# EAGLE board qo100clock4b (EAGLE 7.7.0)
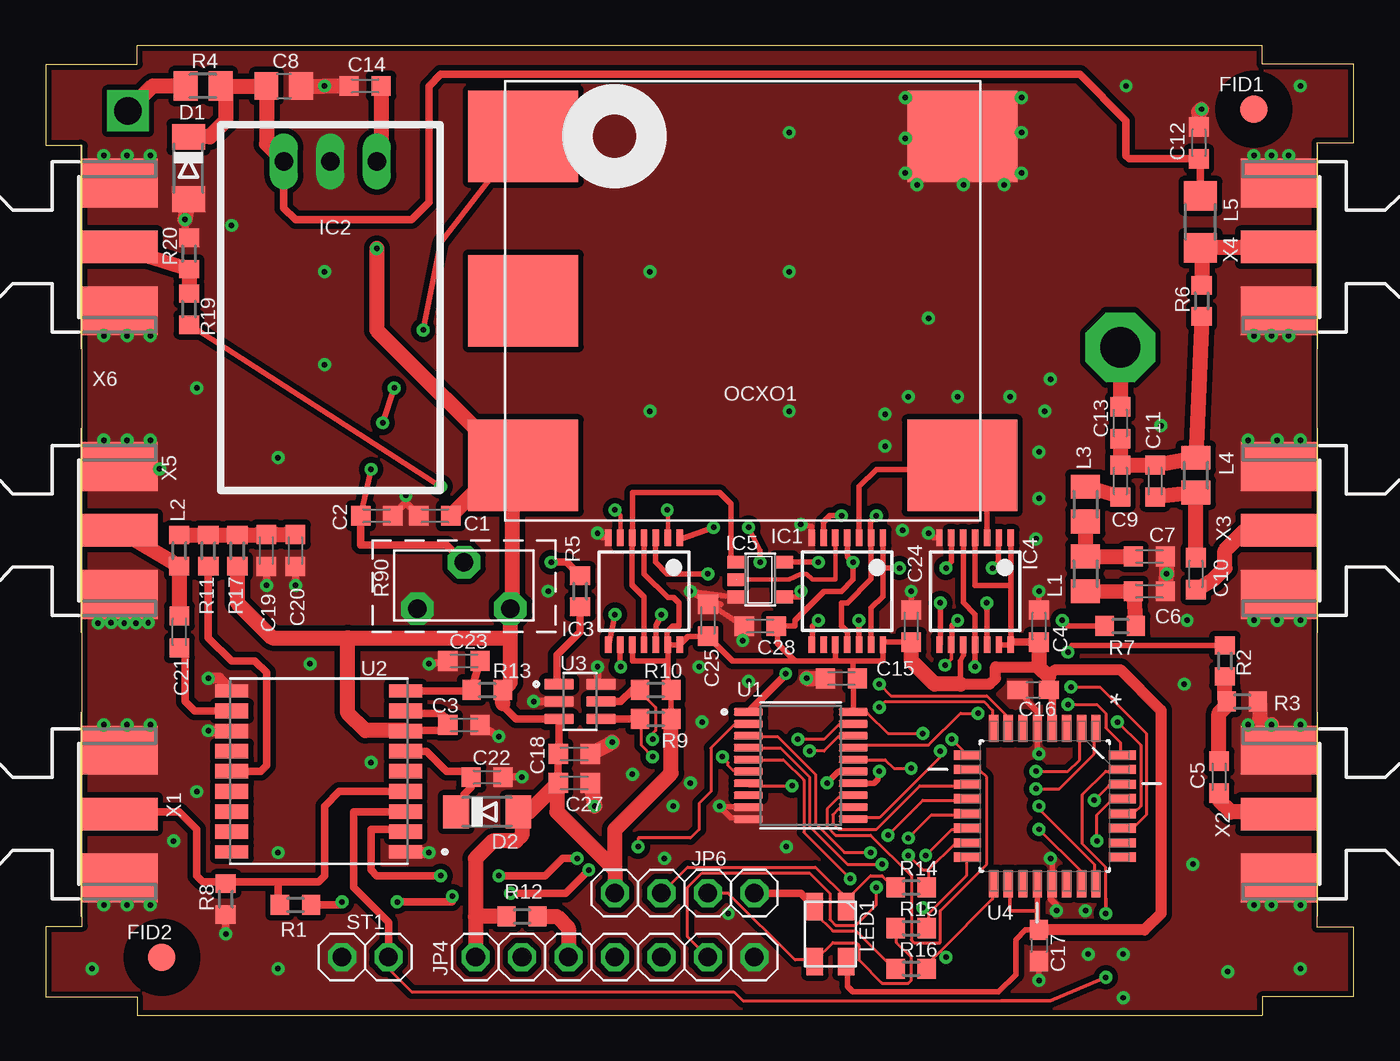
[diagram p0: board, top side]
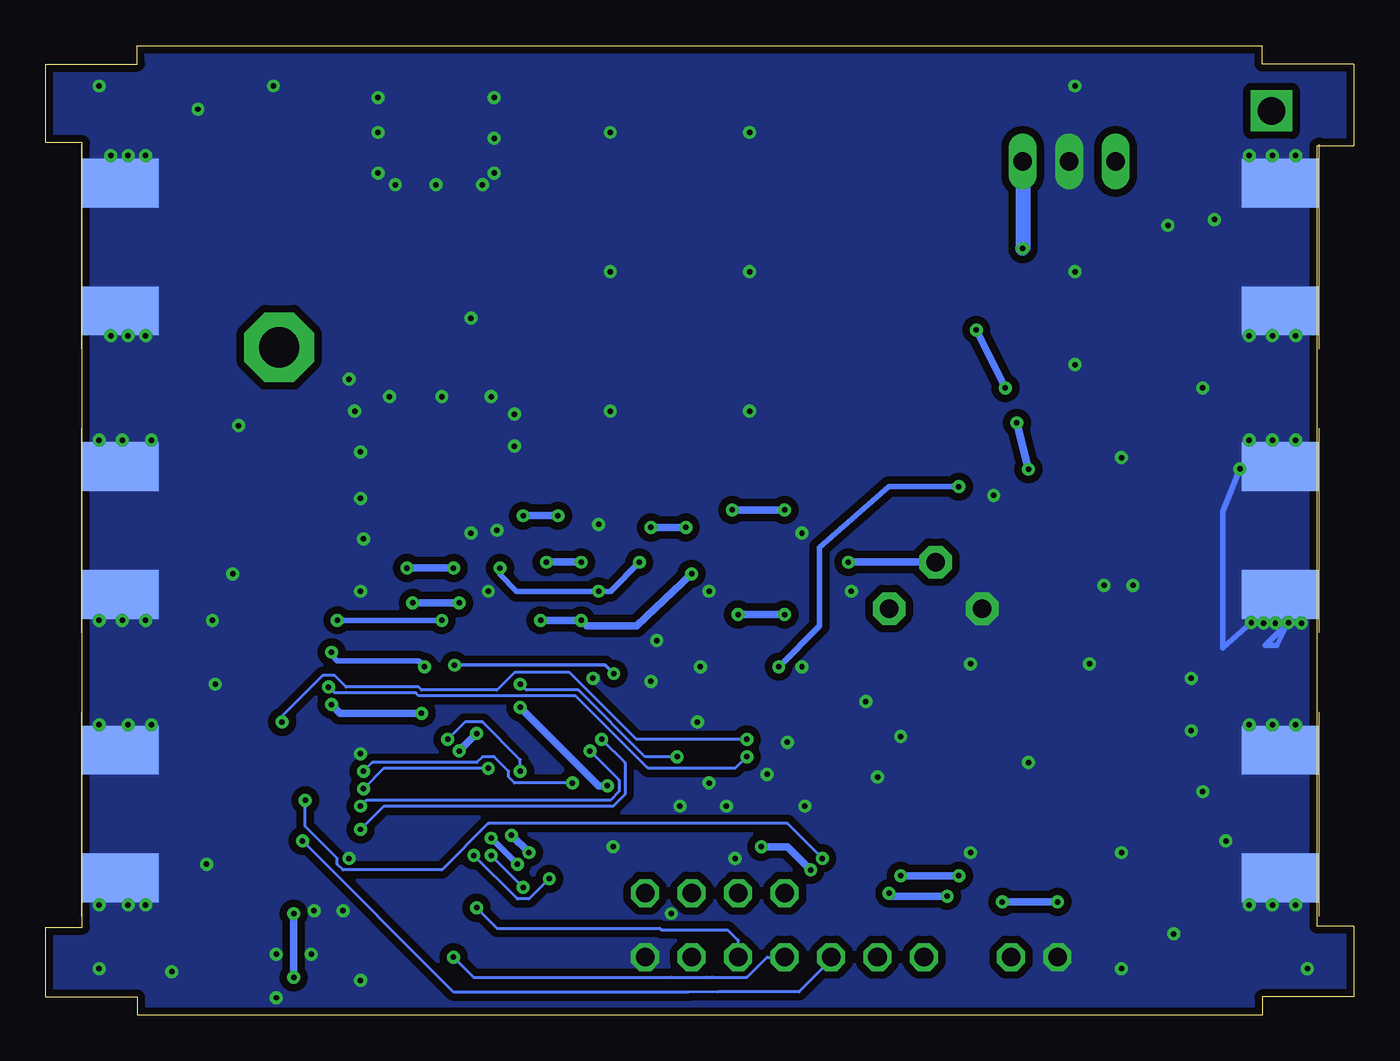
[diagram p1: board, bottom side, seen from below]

Size 71.5 x 53 mm. Coordinates in mm from the lower left corner, seen from the top.
Outline: 5,0 66.5,0 66.5,1 71.5,1 71.5,4.82 69.5,4.82 69.5,47.69 71.5,47.69 71.5,52 66.5,52 66.5,53 5,53 5,52 0,52 0,47.53 2,47.53 2,4.87 0,4.87 0,1 5,1 5,0
Copper layers (1*16): Top 0.035mm / dielectric 1.5mm / Bottom 0.035mm
Design rules "default *": minimum track width 6mil, minimum drill 0.3mm, track to track 6mil, track to pad 6mil, pad to pad 6mil, via to via 6mil, smd to smd 0mil, copper to edge 1mil, drill to drill 8mil, minimum pad ring 10mil, minimum via ring 8mil, stop-mask expansion 4mil, vias tented up to drill 0.51mm, thermal gap 10mil

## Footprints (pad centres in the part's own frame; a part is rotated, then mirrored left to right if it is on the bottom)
C0603K = smd 1.05 x 1.08: 1 -0.875,0; 2 0.875,0
C0805 = smd 1.3 x 1.5: 1 -0.95,0; 2 0.95,0
C0603 = smd 1.1 x 1: 1 -0.85,0; 2 0.85,0
MINIMELF = smd 1.4 x 1.8: A 1.7,0; C -1.7,0
FIDUCIAL = smd 1.5 x 1.5: P$1 0,0
TSSOP14 = smd 0.35 x 0.9: 1 -1.95,-2.925; 2 -1.3,-2.925; 3 -0.65,-2.925; 4 0,-2.925; 5 0.65,-2.925; 6 1.3,-2.925; 7 1.95,-2.925; 8 1.95,2.925; 9 1.3,2.925; 10 0.65,2.925; 11 0,2.925; 12 -0.65,2.925; 13 -1.3,2.925; 14 -1.95,2.925
78SR_SWITCHREG = drill 1.016 long: 1 2.54,0; 2 0,0; 3 -2.54,0
SOT23-5 = smd 0.69 x 0.99: 1 -0.95,-1.29; 2 0,-1.29; 3 0.95,-1.29; 4 0.95,1.3; 5 -0.95,1.3
THICKPIN1,5SQU = drill 1.5 square: P$1 0,0
THICKPIN_OCT = drill 2.2 pad 3.81 octagon: 1 0,0
PINHEAD7X1 = drill 1.016 octagon: 1 -7.62,0; 2 -5.08,0; 3 -2.54,0; 4 0,0; 5 2.54,0; 6 5.08,0; 7 7.62,0
PINHEAD4X1 = drill 1.016 octagon: 1 -5.08,0; 2 -2.54,0; 3 0,0; 4 2.54,0
M0805 = smd 1.3 x 1.6: 1 -0.95,0; 2 0.95,0
R0603 = smd 1 x 1.1: 1 -0.85,0; 2 0.85,0
R1206 = smd 1.6 x 1.803: 1 -1.422,0; 2 1.422,0
PLCC4_WE_LED = smd 1.5 x 0.9: 1 1.51,0.88; 2 1.51,-0.82; 3 -1.49,0.88; 4 -1.49,-0.82
OCXO_2522 = smd 5 x 6: P1 -9,-12; P2 0,-12; P3 9,-12; P4 9,12; P5 -9,12
M2012 = smd 1.3 x 1.6: 1 -0.95,0; 2 0.95,0
MINIPOTI = drill 1.016 pad 1.778 octagon: 1 -2.54,-2.54; 2 2.54,-2.54; 3 0,0
PINHEAD1X2 = drill 1.016 octagon: 1 -1.27,0; 2 1.27,0
SOP65P640X120-20N = smd 1.57 x 0.41: 1 -2.87,2.925; 2 -2.87,2.275; 3 -2.87,1.625; 4 -2.87,0.975; 5 -2.87,0.325; 6 -2.87,-0.325; 7 -2.87,-0.975; 8 -2.87,-1.625; 9 -2.87,-2.275; 10 -2.87,-2.925; 11 2.87,-2.925; 12 2.87,-2.275; 13 2.87,-1.625; 14 2.87,-0.975; 15 2.87,-0.325; 16 2.87,0.325; 17 2.87,0.975; 18 2.87,1.625; 19 2.87,2.275; 20 2.87,2.925
XCVR_MAX-M8C-0 = smd 1.8 x 0.7: 1 -4.75,4.4; 9 -4.75,-4.4; 10 4.75,-4.4; 18 4.75,4.4 | smd 1.8 x 0.8: 2 -4.75,3.3; 3 -4.75,2.2; 4 -4.75,1.1; 5 -4.75,0; 6 -4.75,-1.1; 7 -4.75,-2.2; 8 -4.75,-3.3; 11 4.75,-3.3; 12 4.75,-2.2; 13 4.75,-1.1; 14 4.75,0; 15 4.75,1.1; 16 4.75,2.2; 17 4.75,3.3
SOT95P270X145-6N = smd 1.61 x 0.59: 1 -1.145,0.95; 2 -1.145,0; 3 -1.145,-0.95; 4 1.145,-0.95; 5 1.145,0; 6 1.145,0.95
QFP80P900X900X120-32N = smd 1.473 x 0.508: 1 -4.242,2.794; 2 -4.242,2.007; 3 -4.242,1.194; 4 -4.242,0.406; 5 -4.242,-0.406; 6 -4.242,-1.194; 7 -4.242,-2.007; 8 -4.242,-2.794; 17 4.242,-2.794; 18 4.242,-2.007; 19 4.242,-1.194; 20 4.242,-0.406; 21 4.242,0.406; 22 4.242,1.194; 23 4.242,2.007; 24 4.242,2.794 | smd 0.508 x 1.473: 9 -2.794,-4.242; 10 -2.007,-4.242; 11 -1.194,-4.242; 12 -0.406,-4.242; 13 0.406,-4.242; 14 1.194,-4.242; 15 2.007,-4.242; 16 2.794,-4.242; 25 2.794,4.242; 26 2.007,4.242; 27 1.194,4.242; 28 0.406,4.242; 29 -0.406,4.242; 30 -1.194,4.242; 31 -2.007,4.242; 32 -2.794,4.242
J502-ND-142-0711-821/826 = smd 4.191 x 1.778: 1 2.115,0 | smd 4.191 x 2.667: G@1 2.115,3.495; G@2 2.115,-3.495 | smd 4.191 x 2.667 bottom: G@3 2.115,3.495; G@4 2.115,-3.495

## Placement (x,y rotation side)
C1  100n  [C0603K]  21.27,27.3 180 top
C2  10u  [C0603K]  18.1,27.3 0 top
C3  100n  [C0603K]  22.86,15.88 0 top
C4  100n  [C0603K]  54.29,21.27 90 top
C5  100p  [C0603K]  64.14,13.02 270 top
C6  100p  [C0603K]  60.33,23.18 180 top
C7  100p  [C0603K]  60.33,25.08 180 top
C8  10u  [C0805]  13.02,50.8 0 top
C9  100p  [C0603K]  58.74,29.21 270 top
C10  100n  [C0603K]  62.87,24.13 270 top
C11  100p  [C0603K]  60.64,29.21 90 top
C12  100n  [C0603K]  63.03,47.69 270 top
C13  100p  [C0603K]  58.74,32.38 90 top
C14  10u  [C0603K]  17.46,50.8 180 top
C15  100n  [C0603K]  43.5,18.41 180 top
C16  1u/10  [C0603]  53.98,17.78 180 top
C17  1u/10  [C0603]  54.29,3.81 270 top
C18  100n  [C0603K]  28.89,14.29 0 top
C19  100p  [C0603K]  12.06,25.4 270 top
C20  10u  [C0603K]  13.65,25.4 270 top
C21  100p  [C0603K]  7.3,20.95 270 top
C22  10u  [C0603K]  24.13,13.02 0 top
C23  100n  [C0603K]  22.86,19.37 0 top
C24  100n  [C0603K]  47.31,21.27 90 top
C25  100n  [C0603K]  36.2,21.59 90 top
C27  10u  [C0603K]  28.89,12.7 0 top
C28  100n  [C0603K]  39.05,21.27 0 top
D1  Schottky  [MINIMELF]  7.8,46.31 270 top
D2  Schottky  [MINIMELF]  24.13,11.11 0 top
FID1  FIDUCIAL  [FIDUCIAL]  66.04,49.53 0 top
FID2  FIDUCIAL  [FIDUCIAL]  6.35,3.17 0 top
IC1  74LVC74APW-Q100J  [TSSOP14]  43.81,23.18 180 top
IC2  OKI-78SR-3.3/1.5-W36H-C  [78SR_SWITCHREG]  15.56,46.67 180 top
IC3  74LVC74APW-Q100J  [TSSOP14]  32.7,23.18 180 top
IC4  74LVC74APW-Q100J  [TSSOP14]  50.8,23.18 180 top
IC5  74AHC1G00DBV  [SOT23-5]  39.05,23.81 270 top
JP2  [THICKPIN1,5SQU]  4.49,49.44 90 top
JP3  [THICKPIN_OCT]  58.74,36.51 90 top
JP4  Program  [PINHEAD7X1]  31.11,3.17 0 top
JP6  [PINHEAD4X1]  33.66,6.67 180 top
L1  390nH  [M0805]  56.83,24.13 90 top
L2  47nH  [R0603]  7.3,25.4 90 top
L3  390nH  [M0805]  56.83,27.94 90 top
L4  390nH  [M0805]  62.87,29.53 270 top
L5  4.7uH/1A  [R1206]  63.11,43.37 270 top
LED1  WE:150141M173100  [PLCC4_WE_LED]  42.86,4.45 270 top
OCXO1  ECOC-2522-100.000-3-F-C  [OCXO_2522]  38.1,39.05 270 top
R1  1k  [R0603]  13.65,6.03 180 top
R2  100  [R0603]  64.45,19.37 270 top
R3  100  [R0603]  65.41,17.14 180 top
R4  PTC-fuse 2A  [M2012]  8.61,50.8 0 top
R5  10k  [R0603]  29.21,23.18 90 top
R6  0 Ohms  [R0603]  63.18,39.05 90 top
R7  47  [R0603]  58.74,21.27 0 top
R8  1k  [R0603]  9.84,6.35 90 top
R9  2k2  [R0603]  33.34,16.19 0 top
R10  2k2  [R0603]  33.34,17.78 0 top
R11  10  [R0603]  8.89,25.4 90 top
R12  100k  [R0603]  26.04,5.4 0 top
R13  10k  [R0603]  24.13,17.78 0 top
R14  1k  [R0603]  47.31,6.99 0 top
R15  2k2  [R0603]  47.31,4.76 0 top
R16  2k2  [R0603]  47.31,2.54 0 top
R17  NC  [R0603]  10.48,25.4 90 top
R19  100  [R0603]  7.83,38.6 270 top
R20  100  [R0603]  7.83,41.64 90 top
R90  5k  [MINIPOTI]  22.86,24.77 0 top
ST1  [PINHEAD1X2]  17.46,3.17 0 top
U1  SN74LV8154pwr  [SOP65P640X120-20N]  41.27,13.65 0 top
U2  MAX-8Q  [XCVR_MAX-M8C-0]  14.92,13.34 180 top
U3  MCP4725A0T-E/CH  [SOT95P270X145-6N]  29.21,17.14 0 top
U4  ATMEGA88PB-AU  [QFP80P900X900X120-32N]  54.61,11.43 270 top
X1  SMA  [J502-ND-142-0711-821/826]  1.91,11 0 top
X2  SMA  [J502-ND-142-0711-821/826]  69.53,11 180 top
X3  SMA  [J502-ND-142-0711-821/826]  69.53,26.5 180 top
X4  SMA  [J502-ND-142-0711-821/826]  69.53,42 180 top
X5  GPS-ANT  [J502-ND-142-0711-821/826]  1.91,26.5 0 top
X6  SMA  [J502-ND-142-0711-821/826]  1.91,42 0 top

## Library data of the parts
C1-C25 C27 C28 L1-L5 R1-R17 R19 R20 = rcl
D1 D2 = diode
FID1 FID2 IC2 JP2-JP4 JP6 LED1 R90 ST1 = km
IC1 IC3 IC4 = 74xx-eu
IC5 = 74xx-little-de
OCXO1 = km_HF
U1 = SN74LV8154PWR; AVAILABILITY: In Stock; DESCRIPTION: Dual 16-Bit Binary Counters with 3-State Output Registers 20-TSSOP -40 to 85; MF: Texas Instruments; MP: SN74LV8154PWR; PACKAGE: TSSOP-20 Texas Instruments; PRICE: None; PURCHASE-URL: https://pricing.snapeda.com/search/part/SN74LV8154PWR/?ref=eda
U2 = MAX-M8C-0; AVAILABILITY: In Stock; DESCRIPTION: MAX-M8 RF Receiver BeiDou, Galileo, GLONASS, GNSS, GPS 1.575GHz -167dBm; MF: u-blox; MP: MAX-M8C-0; PACKAGE: SMD-18 u-blox; PRICE: None; PURCHASE-URL: https://pricing.snapeda.com/search/part/MAX-M8C-0/?ref=eda
U3 = MCP4725A0T-E_CH; AVAILABILITY: In Stock; DESCRIPTION: 12 Bit Digital to Analog Converter 1 SOT-23-6; MF: Microchip; MP: MCP4725A0T-E/CH; PACKAGE: SOT-23-6 Microchip; PRICE: None
U4 = atmega48; MPN: ATMEGA48PA-AU; OC_FARNELL: 1715488; OC_NEWARK: 15R0269; PACKAGE: TQFP-32; SUPPLIER: Atmel
X1-X6 = con-coax; MF: JOHNSON COMPONENTS; MPN: 142-0711-821; OC_FARNELL: 1019328; OC_NEWARK: 16F3627

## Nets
+5V: C8.1 C12.2 D1.C IC2.1 L5.1 R4.2
GND: C1.2 C2.2 C3.2 C4.2 C6.1 C7.1 C8.2 C12.1 C14.2 C15.2 C16.2 C17.2 C18.2 C19.2 C20.2 C22.2 C23.1 C24.2 C25.2 C27.2 C28.1 D1.A IC1.7 IC2.2 IC3.7 IC4.7 IC5.3 JP4.7 OCXO1.P5 R3.1 R8.1 R20.2 R90.1 ST1.1 U1.9 U1.10 U2.1 U2.10 U2.12 U3.2 U3.6 U4.5 U4.21 X1.G@1 X1.G@2 X1.G@3 X1.G@4 X2.G@1 X2.G@2 X2.G@3 X2.G@4 X3.G@1 X3.G@2 X3.G@3 X3.G@4 X4.G@1 X4.G@2 X4.G@3 X4.G@4 X5.G@1 X5.G@2 X5.G@3 X5.G@4 X6.G@1 X6.G@2 X6.G@3 X6.G@4
MHZ25: IC4.9 R7.1 U1.1
MHZ100: IC1.3 IC4.3 OCXO1.P4
N$1: C2.1 OCXO1.P1 R5.2 R90.3
N$2: C5.1 R2.2 R3.2
N$3: C5.2 X2.1
N$4: U4.6
N$5: IC4.2 IC4.6
N$6: IC4.8 IC4.12
N$7: IC4.5 IC4.11 R2.1
N$8: R11.1 U2.14
N$9: JP2.P$1 R4.1
N$10: C6.2 L1.1 R7.2
N$11: C7.2 L1.2 L3.1
N$12: C9.2 L3.2
N$13: C10.2 X3.1
N$14: C10.1 C11.1 L4.2
N$15: C9.1 C11.2 C13.1 L4.1 R6.1
N$16: C13.2 JP3.1
N$17: L5.2 R6.2 X4.1
N$18: U1.3 U4.12
N$19: R1.1 U1.2
N$20: C23.2 R13.1 U2.9
N$21: U1.4 U4.13
N$22: U1.5 U4.14
N$23: U1.6 U4.7
N$24: U1.7 U4.8
N$25: IC3.9 R19.2
N$26: R9.1 U3.4 U4.27
N$27: R10.1 U3.5 U4.28
N$28: C19.1 C20.1 L2.2 R11.2 R17.2
N$29: JP6.3 LED1.3 R14.1
N$30: JP6.2 LED1.2 R15.1
N$31: JP6.1 LED1.4 R16.1
N$32: IC1.2 IC1.6 IC1.11
N$33: C21.2 U2.11
N$34: C21.1 L2.1 X5.1
N$35: IC1.8 IC1.12 IC3.3
N$36: C22.1 D2.C U2.6
N$37: IC1.5 IC5.2
N$38: JP4.5 R15.2 U4.16
N$39: JP4.6 R14.2 U4.15
N$40: JP4.4 R16.2 U4.17
N$41: JP4.3 R12.2 U4.29
N$43: IC3.2 IC3.6
N$44: IC3.8 IC3.12
N$45: IC3.5 IC3.11 IC5.1
N$46: IC1.1 IC1.13 IC3.1 IC5.4
N$48: R19.1 R20.1 X6.1
REFCLK: R1.2 R8.2 U2.4 X1.1
RXD: U2.2 U4.30
TXD: ST1.2 U2.3 U4.31
VAL0: U1.19 U4.23
VAL1: U1.18 U4.24
VAL2: U1.17 U4.32
VAL3: U1.16 U4.1
VAL4: U1.15 U4.2
VAL5: U1.14 U4.9
VAL6: U1.13 U4.10
VAL7: U1.12 U4.11
VC: R5.1 U3.1
VCC: C1.1 C3.1 C4.1 C14.1 C15.1 C16.1 C17.1 C18.1 C24.1 C25.1 C27.1 C28.2 D2.A IC1.4 IC1.10 IC1.14 IC2.3 IC3.4 IC3.10 IC3.13 IC3.14 IC4.1 IC4.4 IC4.10 IC4.13 IC4.14 IC5.5 JP4.1 JP6.4 LED1.1 OCXO1.P3 R9.2 R10.2 R12.1 R13.2 R17.1 R90.2 U1.11 U1.20 U2.7 U2.8 U3.3 U4.4 U4.18 U4.20

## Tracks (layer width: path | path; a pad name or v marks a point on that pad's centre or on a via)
+5V
  Top 0.406: IC2.1 13.02,44.13 13.65,43.5 20,43.5 20.95,44.45 20.95,50.8 21.59,51.44 56.52,51.44 59.05,48.9 59.05,46.99 59.23,46.81 C12.2 63.11,46.73 L5.1
  Top 0.813: IC2.1 12.07,47.62 C8.1 R4.2 9.84,50.52 9.84,48.9 8.96,48.02 D1.C
GND  (via drill 0.3)
  Top 0.152: v38.1,20.48 38.26,21.27 C28.1 | v4.45,6.03 4.13,6.35 4.13,7.46 X1.G@2 | v4.45,15.88 4.13,15.56 4.13,14.61 X1.G@3 | 4.13,30 X5.G@3 | v4.45,37.15 4.13,37.47 4.13,38.42 X6.G@2 | v4.45,46.99 4.13,46.67 4.13,45.56 X6.G@3 | v66.99,6.03 67.31,6.35 67.31,7.46 X2.G@3 | X2.G@2 67.31,14.61 67.31,15.72 v66.99,15.88 | v67.31,31.43 67.31,30 X3.G@2 | v66.99,37.15 67.31,37.47 67.31,38.42 X4.G@3 | v66.99,46.99 67.31,46.67 67.31,45.56 X4.G@4
  Top 0.305: v48.26,26.35 48.51,26.1 IC4.7 | v41.27,26.83 41.87,26.71 IC1.7 | v47.31,23.18 C24.2 | v54.29,23.18 C4.2 | v54.29,14.29 54.2,14.38 U4.5 54.2,16.6 53.66,17.14 53.66,17.25 C16.2 | v30.16,26.35 30.41,26.1 IC3.7 | v35.24,23.18 36.91,22.46 C25.2 | v35.24,23.18 37.76,22.84 IC5.3 | v35.24,23.18 38.1,21.27 C28.1 | U1.9 37.41,11.38 v36.83,11.43 37.47,10.79 38.34,10.79 U1.10 | v54.93,8.57 55.02,8.48 U4.21 54.93,7.1 54.93,6.35 55.24,6.03 v55.24,5.71 | C17.2 v54.29,1.91 | X3.G@3 66,23 66,22.5 65.91,21.59 v66.04,21.59 | X5.G@3 4.14,29.87 v6.22,29.87 | v5.6,21.47 5.09,22.76 v4.93,21.43 | X5.G@4 4.04,22.98 v3.58,21.47
  Top 0.406: v50.16,45.4 50.1,45.47 OCXO1.P5 | C19.2 v12.06,23.5 | C20.2 v13.65,23.5 | C2.2 19.68,28.02 | C1.2 19.68,28.02 | 19.68,28.02 v19.68,28.42 | C23.1 v20.95,19.21 | C3.2 v24.77,15.24 | C22.2 v26.04,13.02 | v26.67,17.14 U3.2 | R20.2 7.62,42.7 v7.62,43.5 | R8.1 v9.84,4.45 | U3.6 30.16,18.29 v30.16,19.05
  Top 0.61: U2.1 19.72,8.89 v20.95,8.89 | v8.89,15.56 8.91,15.54 U2.12 | U2.10 9.49,18.41 v8.89,18.41
  Top 0.813: C8.2 v15.24,50.8 C14.2 | v63.18,49.53 63.03,49.37 C12.1 | v7.62,43.5 D1.A | C18.2 v30.96,14.92 | C27.2 v30,11.43 | C7.1 v61.28,24.13 C6.1 | R3.1 66.36,17.04 66.36,16.19 66.67,15.88 v66.99,15.88 | v41.59,18.41 C15.2
  Bottom 0.305: v6.22,29.87 7.16,27.54 7.16,20.07 v5.6,21.47 | v3.58,21.47 4.2,20.23 4.82,20.23 4.02,21.03 X5.G@4
  other vias: 53.34,50.16 53.34,46.04 52.39,45.4 47.62,45.4 46.99,46.04 46.99,50.16 53.34,48.26 46.99,47.94 66.04,46.99 67.94,46.99 66.04,37.15 67.94,37.15 3.17,46.99 5.71,46.99 5.71,37.15 3.17,37.15 3.17,15.88 5.71,15.88 5.71,6.03 3.17,6.03 65.72,31.43 68.58,31.43 67.31,21.59 68.58,21.59 65.72,15.88 68.58,15.88 66.04,6.03 68.58,6.03 3.17,31.43 4.45,31.43 5.71,31.43 2.86,21.43 4.29,21.43 12.7,30.48 15.24,35.56 15.24,40.64 10.16,43.18 8.26,34.29 2.54,2.54 12.7,2.54 33.02,48.26 40.64,48.26 40.64,40.64 33.02,40.64 33.02,33.02 40.64,33.02 48.26,38.1 59.05,50.8 68.58,50.8 68.58,2.54 64.61,2.38 62.23,18.1 14.45,19.21 17.78,13.81 12.7,8.89 35.72,19.05 38.42,18.26 62.39,21.59 54.93,34.77 60.96,32.23 62.71,8.26 33.81,8.57 40.48,9.21 27.46,23.18 8.26,12.22 6.99,9.53 47.15,33.81 49.85,33.81 52.7,33.81 54.61,33.02 54.29,30.8 54.29,28.26 54.13,26.04 45.88,32.86 45.88,31.11 46.83,26.51 34.29,11.43 35.88,16.03 32.07,13.18 35.24,12.7 56.99,3.33 58.9,3.33 58.9,0.95 37.31,5.56 56.83,5.71
  pour Bottom (isolate 0.406, no thermals): 0,0 71.75,0 71.75,53.02 0,53.02
  pour Top (isolate 0.305, no thermals): -0.31,53.52 71.88,53.52 71.88,-0.16 -0.31,-0.16
MHZ25  (via drill 0.3)
  Top 0.152: 57.94,21.27 R7.1
  Top 0.203: 40.45,18.62 v40.45,18.67 | v49.16,19.14 49.5,19.47 IC4.9
  Top 0.305: v49.85,21.59 49.53,21.27 49.53,20.28 IC4.9 49.53,20.22 | v55.56,21.59 55.88,21.27 R7.1
  Top 0.406: U1.1 40.45,18.62
  Bottom 0.203: v40.45,18.67 40.92,19.14 v49.16,19.14
  Bottom 0.305: v49.85,21.59 v55.56,21.59
MHZ100
  Top 0.305: IC4.3 51.45,28.7 OCXO1.P4 49.89,29.84 45.4,29.84 44.47,28.91 IC1.3
N$1  (via drill 0.3)
  Top 0.305: v19.05,34.29 v18.41,32.38 | v17.78,29.84 C2.1 | OCXO1.P1 21.59,42.23 v20.64,37.47
  Top 0.406: R5.2 28.47,24.77 v27.62,24.77 | R90.3 21.91,25.72 17.22,25.72 C2.1
  Bottom 0.406: v27.62,24.77 R90.3 | v20.64,37.47 v19.05,34.29 | v18.41,32.38 v17.78,29.84
N$2
  Top 0.813: C5.1 64.14,16.51 64.56,16.93 R3.2 64.45,17.25 R2.2
N$3
  Top 0.813: X2.1 67.31,11.11 64.77,11.11 64.14,11.75 C5.2
N$5  (via drill 0.3)
  Top 0.305: IC4.2 52.07,26.1 52.07,24.77 v51.75,24.45 | v49.21,24.45 49.5,24.8 IC4.6
  Bottom 0.406: v51.75,24.45 v49.21,24.45
N$6  (via drill 0.3)
  Top 0.305: IC4.8 48.9,20.3 v48.9,22.54 | v51.44,22.54 51.45,22.53 IC4.12
  Bottom 0.406: v48.9,22.54 v51.44,22.54
N$7  (via drill 0.3)
  Top 0.305: IC4.5 50.15,22.56 50.8,21.91 IC4.11 v50.8,19.05 | v55.88,19.84 56.09,20.22 R2.1
  Bottom 0.305: v50.8,19.05 51.12,19.37 55.56,19.37 55.88,19.68 v55.88,19.84
N$8
  Top 0.406: R11.1 8.89,20.64 10.16,19.37 11.43,19.37 12.06,18.73 12.06,13.65 11.75,13.34 U2.14
N$9
  Top 0.813: JP2.P$1 5.85,50.8 R4.1
N$10
  Top 0.813: L1.1 C6.2 R7.2
N$11
  Top 0.813: L3.1 L1.2 C7.2
N$12
  Top 0.813: C9.2 L3.2
N$13
  Top 0.813: C10.2 63.82,23.81 64.45,24.45 64.45,25.4 65.55,26.5 X3.1
N$14
  Top 0.813: C10.1 L4.2 C11.1
N$15
  Top 0.813: C13.1 C9.1 C11.2 L4.1 R6.1
N$16
  Top 0.813: JP3.1 C13.2
N$17
  Top 0.813: X4.1 67.37,41.95 L5.2 63.18,41.88 R6.2
N$18  (via drill 0.3)
  Top 0.152: v46.04,9.84 47.94,11.75 50.32,11.75 U4.12 | v45.09,8.89 43.66,8.89 42.07,10.48 42.07,13.18 40.01,15.24 38.42,15.24 U1.3
  Bottom 0.406: v45.09,8.89 v46.04,9.84
N$19  (via drill 0.3)
  Top 0.152: v32.38,9.21 32.38,9.68 35.24,9.68 35.72,10.16 35.72,11.59 36.35,12.22 36.35,14.61 37.62,15.88 38.26,15.88 U1.2 | 14.61,6.03 R1.1
  Top 0.406: v16.19,6.19 16.03,6.03 R1.1 | v29.69,7.94 28.42,6.67 v25.4,6.67 | v22.23,6.51 22.23,6.19 v19.21,6.19
  Bottom 0.152: v25.4,6.67 25.24,6.51
  Bottom 0.406: v29.69,7.94 30.96,9.21 v32.38,9.21 | v19.21,6.19 v16.19,6.19 | 25.24,6.51 v22.23,6.51
N$20
  Top 0.406: R13.1 23.23,17.73 | 23.23,17.73 U2.9 | 23.23,17.73 23.25,17.71 C23.2
N$21  (via drill 0.3)
  Top 0.152: v47.15,9.68 48.42,10.95 50.32,10.95 U4.13 | v45.72,8.26 43.81,8.26 41.75,10.32 41.75,13.02 40.16,14.61 38.42,14.61 U1.4
  Bottom 0.305: v45.72,8.26 v47.15,9.68
N$22  (via drill 0.3)
  Top 0.152: v48.1,8.73 49.53,10.16 50.32,10.16 U4.14 | v43.97,7.46 41.43,10 41.43,12.86 40.32,13.97 U1.5
  Bottom 0.152: v48.1,8.73 45.72,6.35 45.09,6.35 v43.97,7.46
N$23  (via drill 0.3)
  Top 0.152: v45.56,18.1 46.2,17.46 51.44,17.46 52.55,16.35 52.55,15.72 U4.7 | v36.99,14.13 37.31,13.81 37.31,13.65 37.62,13.34 38.26,13.34 U1.6
  Bottom 0.152: v45.56,18.1 45.24,17.78 42.39,17.78 38.73,14.13 v36.99,14.13
N$24  (via drill 0.3)
  Top 0.152: v45.56,16.83 45.88,17.14 51.28,17.14 51.75,16.67 51.75,15.72 U4.8 | v40.8,12.54 38.42,12.54 U1.7
  Bottom 0.406: v45.56,16.83 41.27,12.54 v40.8,12.54
N$25  (via drill 0.3)
  Top 0.305: IC3.9 31.4,19.08 arc90 v31.43,19.05 | v21.59,28.89 R19.2
  Bottom 0.305: v31.43,19.05 29.21,21.27 29.21,25.56 25.4,28.89 v21.59,28.89
N$26  (via drill 0.3)
  Top 0.152: v56.04,17.94 57.63,17.94 60.17,15.4 60.17,10.95 59.53,10.32 58.9,10.32 U4.27 | v33.18,14.13 32.54,14.76 32.54,16.03 R9.1
  Top 0.406: U3.4 R9.1
  Bottom 0.152: v56.04,17.94 55.72,17.62 51.28,17.62 51.12,17.46 42.55,17.46 38.58,13.49 33.81,13.49 v33.18,14.13
N$27  (via drill 0.3)
  Top 0.152: v58.58,16.03 59.85,14.76 59.85,11.43 59.53,11.11 58.9,11.11 U4.28 | v33.18,15.08 33.18,15.4 33.34,15.56 33.34,16.83 32.54,17.62 R10.1
  Top 0.406: U3.5 31.43,17.14 32.07,17.78 R10.1
  Bottom 0.152: v58.58,16.03 58.58,16.35 56.36,18.57 55.72,18.57 55.09,17.94 51.12,17.94 50.96,17.78 46.83,17.78 45.88,18.73 42.86,18.73 39.21,15.08 v33.18,15.08
N$28
  Top 0.813: L2.2 R11.2 R17.2 arc2 C19.1 arc-4 C20.1
N$29
  Top 0.152: 43.81,6.35 45.09,7.62 45.72,7.62 46.35,6.99 R14.1 | 43.81,6.35 43.81,6.03 LED1.3 43.81,6.35 | 43.81,6.35 42.07,8.1 35.08,8.1 JP6.3
N$30
  Top 0.152: R15.1 46.51,4.76 46.51,3.97 47.31,3.17 47.31,1.91 47.15,1.75 45.72,1.75 44.45,3.02 44.45,3.81 44.29,3.97 43.02,3.97 42.07,3.02 LED1.2 41.91,3.02 40.96,3.02 37.31,6.67 JP6.2
N$31
  Top 0.152: R16.1 46.35,2.54 44.29,4.6 43.02,4.6 42.07,5.56 42.07,5.87 LED1.4 41.91,6.03
  Top 0.406: JP6.1 41.27,6.67 41.91,6.03
N$32  (via drill 0.3)
  Top 0.305: IC1.11 43.81,20.95 43.5,21.27 43.5,22.54 43.81,22.54 45.12,23.84 IC1.2 45.09,26.13 45.09,26.99 v45.4,27.3 | v43.5,27.3 42.86,27.3 42.52,26.96 IC1.6
  Bottom 0.406: v45.4,27.3 v43.5,27.3
N$33
  Top 0.406: C21.2 7.62,20.08 7.62,17.14 8.13,16.64 U2.11
N$34
  Top 0.813: X5.1 L2.1 C21.1
N$35  (via drill 0.3)
  Top 0.305: IC1.8 41.91,20.3 41.91,21.27 v42.23,21.59 | v44.45,21.59 44.47,21.57 IC1.12 | IC3.3 33.34,26.09 33.34,24.77 33.97,24.13 v36.2,24.13
  Bottom 0.406: v44.45,21.59 v42.23,21.59 41.91,21.27 39.21,21.27 v36.2,24.13
N$36
  Top 0.406: U2.6 20.81,14.44 21.91,13.34 22.94,13.34 C22.1 23.25,12.46 22.86,12.06 22.86,11.54 D2.C
N$37
  Top 0.254: IC5.2 40.64,23.81 41.27,24.13 41.59,24.13 41.91,23.81 43.18,23.81 IC1.5
N$38  (via drill 0.3)
  Top 0.152: 48.26,5.56 48.26,4.76 R15.2 | 48.26,5.56 50.32,7.62 50.32,8.57 U4.16 | 48.26,5.56 v47.94,5.87
  Bottom 0.152: v47.94,5.87 46.83,4.76 37.94,4.76 37.85,4.67 34.23,4.67 33.66,4.1 JP4.5
N$39  (via drill 0.3)
  Top 0.152: 48.26,7.94 48.26,6.99 R14.2 | 48.26,7.94 49.69,9.37 50.32,9.37 U4.15 | 48.26,7.94 47.94,7.94 v47.15,8.73 | v45.4,6.99 45.4,6.03 44.29,4.92 43.18,4.92 42.86,5.24 42.86,6.67 41.75,7.78 35.88,7.78 35.08,6.99 35.08,4.29 JP4.6
  Bottom 0.152: v45.4,6.99 v47.15,8.73
N$40  (via drill 0.3)
  Top 0.152: 48.9,3.49 51.75,6.35 51.75,7.14 U4.17 | 48.9,3.49 48.26,2.86 48.26,2.54 R16.2 | 48.9,3.49 v49.21,3.17
  Bottom 0.152: JP4.4 32.07,3.17 33.17,2.07 33.34,2.06 34.29,2.06 35.08,2.08 35.4,2.08 35.88,2.06 36.83,2.06 37.31,2.07 37.78,2.06 48.1,2.06 v49.21,3.17
N$41  (via drill 0.3)
  Top 0.152: v57.47,9.53 57.47,10.95 58.26,11.75 58.74,11.75 U4.29
  Top 0.813: R12.2 27.94,5.4 28.57,4.76 JP4.3
  Bottom 0.152: v57.47,9.53 49.2,1.25 36.34,1.25 34.77,1.27 30.32,1.27 28.57,3.02 JP4.3
N$43  (via drill 0.3)
  Top 0.254: IC3.6 31.43,26.13 31.43,27.3 v31.11,27.62 | v33.97,27.62 34,27.59 IC3.2
  Bottom 0.406: v31.11,27.62 v33.97,27.62
N$44  (via drill 0.3)
  Top 0.305: IC3.8 30.8,20.3 v31.11,21.91 | v33.66,21.91 33.35,21.29 IC3.12
  Bottom 0.406: v31.11,21.91 v33.66,21.91
N$45
  Top 0.305: IC3.11 32.7,22.86 32.05,23.51 IC3.5 32.07,26.12 32.07,28.57 36.83,28.57 37.47,27.94 37.47,25.06 IC5.1
N$46  (via drill 0.3)
  Top 0.305: 45.77,24.45 45.77,22.91 45.12,22.25 IC1.13 | 45.77,24.45 IC1.1 | IC5.4 41.27,22.86 v41.27,23.18 | v46.67,24.45 45.77,24.45 | IC3.1 34.72,26.04 v36.51,26.67 | v38.42,26.67 39.05,25.4 v39.05,24.77
  Bottom 0.305: v46.67,24.45 46.67,24.09 45.77,23.18 v41.27,23.18 40.64,23.18 v39.05,24.77
  Bottom 0.406: v36.51,26.67 v38.42,26.67
N$48
  Top 0.813: X6.1 R20.1 R19.1
REFCLK
  Top 0.406: X1.1 4.02,11.11 7.3,11.11 8.26,10.16 8.26,7.62 8.57,7.3 9.74,7.3 | 9.74,7.3 12.7,7.3 | 12.7,7.3 14.92,7.3 15.24,7.62 15.24,11.43 16.05,12.23 U2.4 | R8.2 9.74,7.3 | R1.2 12.7,6.13 12.7,7.3
RXD  (via drill 0.3)
  Top 0.152: v57.31,11.75 58.1,12.54 58.74,12.54 U4.30
  Top 0.406: U2.2 19.55,10.16 17.78,10.16 17.78,7.94 18.1,7.62 v21.59,7.62 | v24.77,7.62 27.3,7.62 28.26,8.57 v29.05,8.57
  Bottom 0.152: v57.31,11.75 57.31,10.32 55.56,8.57 55.56,8.26 55.24,7.94 49.85,7.94 47.31,10.48 30.96,10.48 v29.05,8.57
  Bottom 0.406: v21.59,7.62 v24.77,7.62
TXD  (via drill 0.3)
  Top 0.152: 57.94,6.35 57.94,8.1 56.67,9.37 56.67,12.06 57.94,13.34 58.74,13.34 U4.31 | 52.23,0.79 38.1,0.79 37.62,1.28 36.99,1.27 20,1.27 18.73,2.54 ST1.2 | 16.83,6.83 16.91,6.91
  Top 0.203: 57.94,6.35 v57.94,5.56 | v57.94,2.06 54.93,0.79 52.23,0.79
  Top 0.406: U2.3 19.65,11.11 16.83,11.11 16.83,6.99 16.91,6.91 18.73,5.08 ST1.2
  Bottom 0.406: v57.94,5.56 v57.94,2.06
VAL0  (via drill 0.3)
  Top 0.152: v54.29,10.16 56.52,7.94 56.52,7.3 U4.23 | v41.12,15.08 42.55,15.08 43.34,15.88 44.13,15.88 U1.19
  Bottom 0.152: v54.29,10.16 53.02,11.43 40.48,11.43 39.85,12.06 39.85,13.81 v41.12,15.08
VAL1  (via drill 0.3)
  Top 0.152: v54.29,11.43 54.29,11.27 57.31,8.26 57.31,7.3 U4.24 | v41.75,14.45 42.55,14.45 43.34,15.24 44.13,15.24 U1.18
  Bottom 0.152: v54.29,11.43 53.98,11.75 40.64,11.75 40.16,12.22 40.16,12.86 v41.75,14.45
VAL2  (via drill 0.3)
  Top 0.152: v55.88,16.99 57.47,16.99 57.94,16.51 57.94,15.72 58.74,14.92 58.74,14.29 U4.32 | v50.96,16.51 50.01,16.51 48.26,14.76 44.29,14.76 U1.17
  Bottom 0.406: v55.88,16.99 55.4,16.51 v50.96,16.51
VAL3  (via drill 0.3)
  Top 0.152: v54.13,12.38 55.4,12.38 57.31,14.29 57.31,15.56 U4.1 | v47.31,13.49 46.35,13.49 45.88,13.97 44.29,13.97 U1.16
  Bottom 0.152: v54.13,12.38 53.02,13.49 v47.31,13.49
VAL4  (via drill 0.3)
  Top 0.152: v54.13,13.34 55.88,13.34 56.52,13.97 56.52,15.56 U4.2
  Top 0.305: v42.7,12.7 43.33,13.33 U1.15
  Bottom 0.152: v54.13,13.34 53.66,13.81 47.94,13.81 47.62,14.13 46.99,14.13 46.2,13.34 46.2,13.02 45.88,12.7 v42.7,12.7
VAL5  (via drill 0.3)
  Top 0.152: v49.53,15.08 50.32,14.29 U4.9 | 44.29,12.7 U1.14
  Top 0.305: v45.56,13.34 45.5,13.27 45.5,12.9 45.28,12.68 U1.14
  Bottom 0.152: v49.53,15.08 48.58,16.03 47.62,16.03 45.56,13.97 v45.56,13.34
VAL6
  Top 0.152: U4.10 50.48,13.34 51.12,13.34 51.44,13.02 51.44,8.26 48.9,5.71 48.9,3.97 47.47,3.97 47.31,4.13 47.31,7.62 45.09,9.84 43.18,9.84 42.7,10.32 42.7,11.27 43.34,11.91 44.13,11.91 U1.13
VAL7
  Top 0.152: U4.11 50.32,12.54 47.78,12.54 45.4,10.16 43.34,10.16 43.02,10.48 43.02,10.95 43.34,11.27 44.13,11.27 U1.12
VC
  Top 0.406: U3.1 27.94,18.22 27.94,19.68 29.21,20.95 R5.1
VCC  (via drill 0.3)
  Top 0.152: v48.9,14.45 48.9,14.13 45.56,10.79 44.29,10.79 U1.11 | v47.94,15.4 46.04,15.4 44.93,16.51 44.29,16.51 U1.20
  Top 0.203: U4.18 52.7,7.19 52.7,5.71 54.2,5.71 54.2,5.4 | U4.4 54.93,15.67 | 54.83,18.52 C16.1
  Top 0.305: IC4.14 52.75,23.5 | 52.75,23.5 IC4.1 | IC4.4 50.8,23.5 52.75,23.5 | IC4.14 IC4.13 52.07,20.22 | IC4.14 52.9,20.4 | IC1.10 43.18,20.24 43.18,19.37 | 43.18,19.37 44.13,19.37 | 44.13,19.37 45.72,19.37 45.77,19.41 IC1.14 45.91,20.4 C24.1 47.31,19.05 | IC5.5 v42.23,24.77 | IC1.4 43.81,25.08 v44.13,24.77 44.13,23.81 43.5,23.18 42.55,23.18 40.96,21.59 40.96,21.27 C28.2 40.01,21.2 40.01,20.32 40.96,19.37 | 40.96,19.37 43.18,19.37 | 40.96,19.37 37.54,19.37 C25.1 35.12,20.71 IC3.14 IC3.13 | R9.2 R10.2 34,17.96 34,19.37 | 34,19.37 IC3.13 | IC3.4 32.7,24.13 34,22.83 34.32,22.83 34.61,22.54 34.61,21.27 34.29,21.27 33.97,20.95 33.97,20.28 IC3.13 | IC3.10 32.07,20.24 32.07,19.37 34,19.37 | IC4.10 50.16,20.24 50.16,19.68 50,19.37 50,18.1 | U4.20 54.2,5.4 54.2,4.75 C17.1 53.55,4.66 53.02,4.13 53.02,2.22 52.07,1.27 44.13,1.27 43.81,1.59 43.81,2.86 LED1.1 | 44.13,19.37 44.13,18.66 C15.1 44.15,18.19 U1.20
  Top 0.406: C27.1 C18.1 28.07,14.34 U3.3 25.71,16.2 25.08,16.83 25.08,17.88 25.4,18.2 | U2.8 19.8,16.51 21.35,16.51 arc-90 C3.1 arc-90 21.67,15.56 19.65,15.56 | 52.9,20.4 C4.1 | C16.1 55.02,17.59 U4.4
  Top 0.61: 50,18.1 51.59,18.1 51.91,18.41 51.91,19.05 54.29,19.05 | 54.83,18.52 55.2,18.89 58.74,18.89 60.96,16.67 60.96,5.56 60.06,4.66 C17.1
  Top 0.813: C14.1 18.34,46.91 IC2.3 | 31.11,7.94 27.94,11.11 27.94,12.62 C27.1 26.43,11.11 D2.A 26.04,10.91 26.04,9.84 25.72,9.53 24.45,9.53 23.5,8.57 23.5,5.4 | v18.1,41.91 18.1,37.47 25.51,30.05 | 25.51,30.05 OCXO1.P3 | C1.1 24.89,30.05 25.51,30.05 | 25.51,30.05 25.51,22.34 R90.2 25.4,20.64 | 25.4,20.64 25.4,18.2 R13.2 24.98,17.04 | R17.1 10.48,22.54 12.38,20.64 16.51,20.64 | 16.51,20.64 25.4,20.64 | 31.11,7.94 31.11,10.16 34.19,13.23 R9.2 | 31.11,7.94 JP6.4 | U2.7 19.65,15.56 17.46,15.56 16.51,16.51 16.51,20.64 | 23.5,5.4 JP4.1 | R12.1 23.5,5.4 | 50,18.1 48.58,18.1 47.31,19.37 C24.1 | C4.1 54.29,19.05 54.83,18.52
  Bottom 0.406: v42.23,24.77 v44.13,24.77 | v47.94,15.4 v48.9,14.45
  Bottom 0.813: IC2.3 v18.1,41.91

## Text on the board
Document: DJ0ABR | VC | +12V | GND | 25MHz | OCXO | QO-100 / Clock / Center / V.4b | LNB | 10MHz | 3v3 | 100MHz | GPS | adj. | RX | ANT | GPS | * | * | * | 50MHz | 3v3 | REF | CLK | 3v3 | GND | GND | TxD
